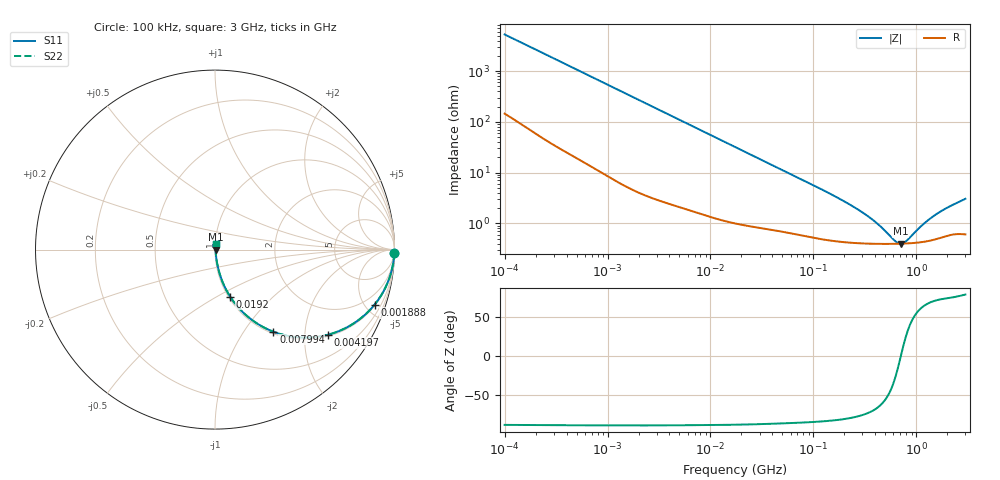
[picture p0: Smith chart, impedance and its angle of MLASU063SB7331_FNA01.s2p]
! MLASU063SB7331_FNA01  S-PARAMETER MODEL  ( Standard Model )
! Model Generated by TAIYO YUDEN Corporation (http://www.ty-top.com)
! Version 1.0
! TAIYO YUDEN Control No. 220601
! Copyright(c) 2012 TAIYO YUDEN CO.,LTD. All Rights Reserved.
! Product Description (link to TY-COMPAS)
! https://ds.yuden.co.jp/TYCOMPAS/or/detail?pn=MLASU063SB7331KFNA01&u=M
! Products Name : Multilayer Ceramic Capacitors
! Characteristics :
!  Capacitance : 330 [pF] , Rated Voltage : 50 [V] , TCC : X7R
!  Case Size : 0.6 x 0.3 / 0.024 x 0.012 [mm/inch] , Thickness : 0.3 / 0.012 [mm/inch]
!  (Conditions: Temperature = 25 [degC] , DC Bias Voltage = 0 [V])
! External Node Assignments :
!  1  o---| |---o  2
! GND o---------o GND
! Frequency Range : 100kHz  -  3GHz  [ 401 STEP ]
# MHZ S RI R 50
! Freq[MHz].  S11 Real  S11 Imag  S21 Real  S21 Imag  S12 Real  S12 Imag  S22 Real  S22 Imag
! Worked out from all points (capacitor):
!   401 points, 100 kHz to 3 GHz, reference 50 ohm
!   read as one part in series: C = 301 pF near 105.3 kHz
!   lowest |Z| = 397 mohm at 708.5 MHz (marker M1)
!   series resonance near 708.5 MHz, so ESL is about 170 pH
!   S11 on the Smith chart (normalised r, x): 100 kHz: open; 1.888 MHz: 1.08, -5.76; 4.197 MHz: 1.05, -2.60; 7.994 MHz: 1.03, -1.38; 19.2 MHz: 1.02, -0.58; 3 GHz: 1.01, +0.06
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0.1  0.9991 -0.019  0.000884 0.019  0.000884 0.019  0.9991 -0.019
0.562235  0.9874 -0.1029  0.0126 0.1029  0.0126 0.1029  0.9874 -0.1029
1.127518  0.9557 -0.1982  0.0443 0.1982  0.0443 0.1982  0.9557 -0.1982
1.887902  0.8888 -0.3071  0.1112 0.3071  0.1112 0.3071  0.8888 -0.3071
3.161081  0.7451 -0.4278  0.2549 0.4278  0.2549 0.4278  0.7451 -0.4278
4.197169  0.6269 -0.4748  0.3731 0.4748  0.3731 0.4748  0.6269 -0.4748
5.718342  0.4794 -0.4897  0.5206 0.4897  0.5206 0.4897  0.4794 -0.4897
7.994228  0.325 -0.4574  0.675 0.4574  0.675 0.4574  0.325 -0.4574
11.76708  0.1867 -0.377  0.8133 0.377  0.8133 0.377  0.1867 -0.377
17.7727  0.0959 -0.2791  0.9041 0.2791  0.9041 0.2791  0.0959 -0.2791
19.20135  0.0843 -0.2619  0.9157 0.2619  0.9157 0.2619  0.0843 -0.2619
40.54368  0.0256 -0.1334  0.9744 0.1334  0.9744 0.1334  0.0256 -0.1334
97.38194  0.00849 -0.0569  0.9915 0.0569  0.9915 0.0569  0.00849 -0.0569
294.964  0.00427 -0.0162  0.9957 0.0162  0.9957 0.0162  0.00427 -0.0162
412.3589  0.00401 -0.00926  0.996 0.00926  0.996 0.00926  0.00401 -0.00926
547.5153  0.00393 -0.00425  0.9961 0.00425  0.9961 0.00425  0.00393 -0.00425
639.0768  0.00393 -0.00169  0.9961 0.00169  0.9961 0.00169  0.00393 -0.00169
708.4746  0.00395 3.25e-07  0.996 -3.25e-07  0.996 -3.25e-07  0.00395 3.25e-07
805.9132  0.004 0.00211  0.996 -0.00211  0.996 -0.00211  0.004 0.00211
1156.079  0.00434 0.00832  0.9957 -0.00832  0.9957 -0.00832  0.00434 0.00832
1535  0.00501 0.0138  0.995 -0.0138  0.995 -0.0138  0.00501 0.0138
3000  0.00688 0.0294  0.9931 -0.0294  0.9931 -0.0294  0.00688 0.0294
